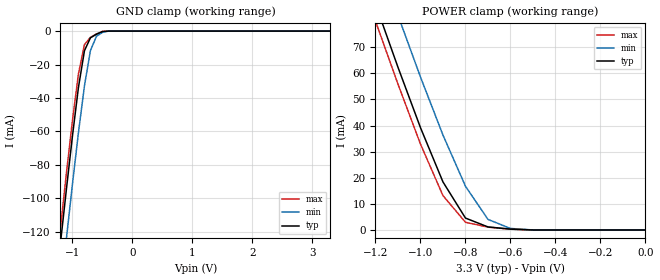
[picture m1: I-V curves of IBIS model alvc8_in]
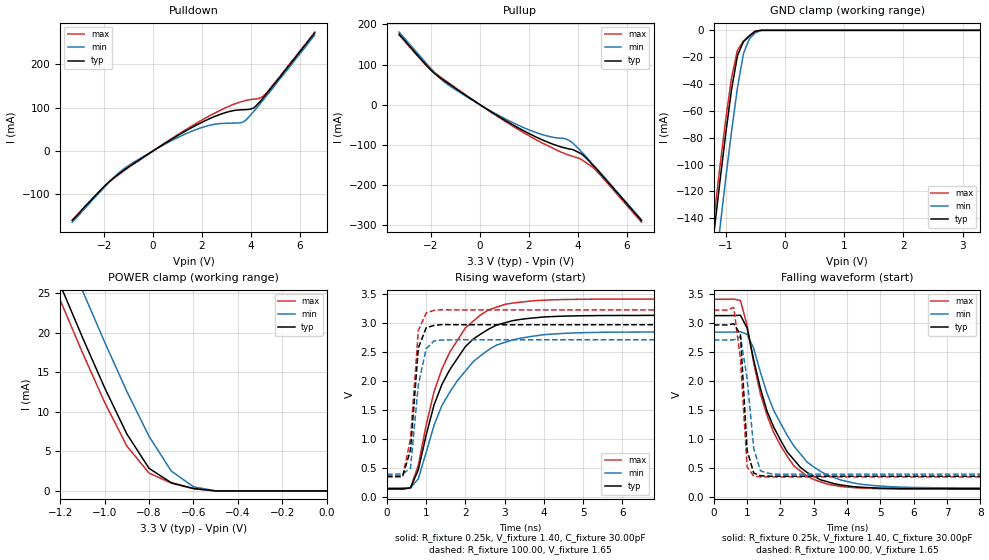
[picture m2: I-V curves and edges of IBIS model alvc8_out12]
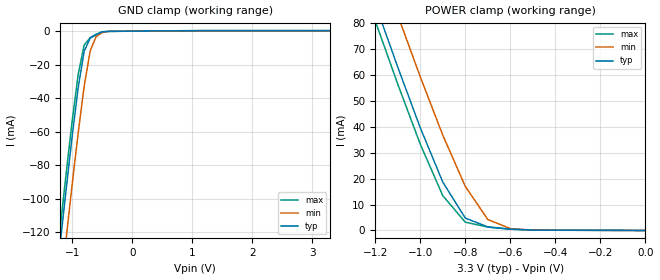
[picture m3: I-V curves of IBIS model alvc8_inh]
| IBIS file 162244ah.ibs created by s2ibis2 version 1.1
| North Carolina State University Electronics Research Laboratory  1995
[IBIS ver]   2.1
[File name]   162244ah.ibs
[File Rev]   1.0
[Date]   03/01/99 rtk rtk
[Source]   Integrated Device Technology, Inc.
[Notes]   1.Temperatures: typ=25C, min=100C, max=0C 2.RRmp rates based
   on 50 ohm load.
[Disclaimer] Integrated Device Technology, Inc. ("IDT") hereby grants the
   user of this IBIS model a non-exclusive, nontransferable
   license to use this IBIS model under the following terms. The
   user is granted this license only to use the IBIS model and is
   not granted rights to sell, copy (except as needed to run the
   IBIS model), rent, lease or sub-license the IBIS model in
   whole or in part, or in modified form to anyone. The User may
   modify the IBIS model to suit its specific applications, but
   rights to derivative works and such modifications shall belong
   to IDT. This IBIS model is provided on an AS IS" basis and IDT
   makes absolutely no warranty with respect to the information
   contained herein. IDT DISCLAIMS AND CUSTOMER WAIVES ALL
   WARRANTIES, EXPRESS AND IMPLIED, INCLUDING WARRANTIES OF
   MERCHANTABILITY AND FITNESS FOR A PARTICULAR PURPOSE. THE
   ENTIRE RISK AS TO QUALITY AND PERFORMANCE IS WITH THE USER
   ACCORDINGLY, IN NO EVENT SHALL IDT BE LIABLE FOR ANY DIRECT OR
   INDIRECT DAMAGES, WHETHER IN CONTRACT OR TORT, INCLUDING ANY
   LOST PROFITS OR OTHER INCIDENTAL, CONSEQUENTIAL, EXEMPLARY, OR
   PUNITIVE DAMAGES ARISING OUT OF THE USE OR APPLICATION OF THE
   IBIS model. Further, IDT reserves the right to make changes
   without notice to any product herein to improve reliability,
   function, or design. IDT does not convey any license under
   patent rights or any other intellectual property rights,
   including those of third parties. IDT is not obligated to
   provide maintenance or support for the licensed IBIS model.
[Copyright]   Copyright 1997, Integrated Device Technology, Inc. all rights
   reserved
|   Component ALVCH 162244
[Component]   ALVCH162244
[Manufacturer]   Integrated Device Technology
[Package]
| PA48
| variable   typ   min   max
R_pkg   6.50m   5.00m   10.00m
L_pkg   3.20nH   2.50nH   4.40nH
C_pkg   0.27pF   0.01pF   0.98pF
| PV48   typ   min   max
|R_pkg   6.5m   5.00m   10.00m
|L_pkg   4.75nH   3.82nH   6.72nH
|C_pkg   0.24pF   0.01pF   1.55pF
[Pin]  signal_name   model_name   R_pin   L_pin   C_pin
1   1OEB   alvc8_in
2   1Y1   alvc8_out12
3   1Y2   alvc8_out12
4   GND   GND
5   1Y3   alvc8_out12
6   1Y4   alvc8_out12
7   VCC   POWER
8   2Y1   alvc8_out12
9   2Y2   alvc8_out12
10   GND   GND
11   2Y3   alvc8_out12
12   2Y4   alvc8_out12
13   3Y1   alvc8_out12
14   3Y2   alvc8_out12
15   GND   GND
16   3Y3   alvc8_out12
17   3Y4   alvc8_out12
18   VCC   POWER
19   4Y1   alvc8_out12
20   4Y2   alvc8_out12
21   GND   GND
22   4Y3   alvc8_out12
23   4Y4   alvc8_out12
24   4OEB   alvc8_in
25   3OEB   alvc8_in
26   4A4   alvc8_inh
27   4A3   alvc8_inh
28   GND   GND
29   4A2   alvc8_inh
30   4A1   alvc8_inh
31   VCC   POWER
32   3A4   alvc8_inh
33   3A3   alvc8_inh
34   GND   GND
35   3A2   alvc8_inh
36   3A1   alvc8_inh
37   2A4   alvc8_inh
38   2A3   alvc8_inh
39   GND   GND
40   2A2   alvc8_inh
41   2A1   alvc8_inh
42   VCC   POWER
43   1A4   alvc8_inh
44   1A3   alvc8_inh
45   GND   GND
46   1A2   alvc8_inh
47   1A1   alvc8_inh
48   2OEB   alvc8_in
| Models and submodels in the file (3): alvc8_in (Input), alvc8_out12 (3-state), alvc8_inh (Input)
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| in   in   dummy_model
| oe   oe   dummy_model
|   Model alvc8_in
[Model]   alvc8_in
Model_type   Input
Vinl =  0.800V
Vinh =  2.000V
C_comp   3.00pF   NA   NA
[Temperature Range]   25.00   100.00   0.000
[Voltage Range]   3.30V   3.00V   3.60V
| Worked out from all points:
|   GND clamp passes 1 mA (typ) near -0.54 V on its own axis
|   POWER clamp passes 1 mA (typ) near -0.68 V on its own axis
[GND_clamp]
| voltage   I(typ)   I(min)   I(max)
-3.3V     -860mA     -887mA     -851mA
-1.3V     -161mA     -190mA     -151mA
-1.2V     -127mA     -157mA     -118mA
-1.1V     -94.41mA   -124mA     -84.85mA
-1V       -62.78mA   -91.54mA   -53.52mA
-900mV    -33.71mA   -60.78mA   -25.6mA
-800mV    -11.74mA   -32.83mA   -8.09mA
-700mV    -4.033mA   -11.65mA   -3.7mA
-600mV    -1.899mA   -3.108mA   -1.699mA
-500mV    -308uA     -810uA     -172uA
-400mV    -3.848nA   -9.872uA   -399pA
3.3V      39.6pA     19.33nA    26.4pA
[POWER_clamp]
| voltage   I(typ)   I(min)   I(max)
-3.3V     630mA      648mA      624mA
-1.2V     86.56mA    106mA      80.02mA
-1.1V     62.33mA    82.22mA    55.88mA
-1V       39.2mA     58.61mA    32.91mA
-900mV    18.4mA     36.35mA    13.15mA
-800mV    4.556mA    16.76mA    2.954mA
-700mV    1.164mA    4.056mA    1.087mA
-600mV    320uA      578uA      299uA
-500mV    40.08nA    12.23uA    3.465nA
0V        39.6pA     59.11pA    43.2pA
|   Model alvc8_out12
[Model]   alvc8_out12
Model_type   3-state
Polarity   Non-Inverting
Enable   Active-High
Vmeas =  1.500V
C_comp   3.00pF   NA   NA
[Temperature Range]   25.00   100.00   0.000
[Voltage Range]   3.30V   3.00V   3.60V
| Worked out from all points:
|   slope of the pulldown table from 0 to 0.495 V, typ, clamps not added: 27.6 ohm
|   slope of the pullup table from 0 to 0.495 V, typ, clamps not added: 25.8 ohm
|   GND clamp passes 1 mA (typ) near -0.51 V on its own axis
|   POWER clamp passes 1 mA (typ) near -0.69 V on its own axis
|   rising waveform, R_fixture 0.25k, V_fixture 1.40, C_fixture 30.00pF: 20-80 % time 1.05ns typ, 1.2ns min, 980ps max; typ from 0.138 V to 3.12 V
|   rising waveform, R_fixture 100.00, V_fixture 1.65: 20-80 % time 178ps typ, 250ps min, 201ps max; typ from 0.356 V to 2.96 V
|   falling waveform, R_fixture 0.25k, V_fixture 1.40, C_fixture 30.00pF: 20-80 % time 1.12ns typ, 1.35ns min, 1.05ns max; typ from 3.12 V to 0.138 V
|   falling waveform, R_fixture 100.00, V_fixture 1.65: 20-80 % time 157ps typ, 252ps min, 217ps max; typ from 2.96 V to 0.356 V
[Pulldown]
| voltage   I(typ)   I(min)   I(max)
-3.3V     -161mA     -165mA     -160mA
-1.8V     -71.5mA    -73.3mA    -72.6mA
-1.3V     -49.1mA    -46.1mA    -50.8mA
-600mV    -22.1mA    -19.8mA    -23.1mA
800mV     28.5mA     25mA       30mA
1.9V      63.5mA     52.4mA     68.3mA
3V        89.4mA     63.9mA     101mA
3.7V      95.4mA     67.5mA     115mA
4.1V      99.1mA     90.7mA     120mA
4.4V      116mA      111mA      123mA
4.6V      130mA      125mA      132mA
6.6V      273mA      268mA      275mA
[Pullup]
| voltage   I(typ)   I(min)   I(max)
-3.3V     176mA      181mA      174mA
-1.9V     80.3mA     83.6mA     82mA
-1.5V     61.8mA     58.9mA     64.3mA
-1V       40.8mA     37.7mA     42.5mA
400mV     -15.6mA    -14.2mA    -16.4mA
1.7V      -62.2mA    -54.9mA    -66.6mA
2.9V      -96.6mA    -80.2mA    -106mA
3.5V      -108mA     -85.3mA    -123mA
3.8V      -112mA     -96mA      -129mA
4.2V      -125mA     -121mA     -139mA
4.7V      -156mA     -155mA     -161mA
6.6V      -289mA     -287mA     -293mA
[GND_clamp]
| voltage   I(typ)   I(min)   I(max)
-3.3V     -1.007A    -1.04A     -997mA
-1.3V     -191mA     -226mA     -180mA
-1.2V     -152mA     -187mA     -141mA
-1.1V     -114mA     -149mA     -103mA
-1V       -77.54mA   -111mA     -67.03mA
-900mV    -44.06mA   -75.31mA   -35.25mA
-800mV    -18.73mA   -42.66mA   -14.81mA
-700mV    -8.526mA   -17.61mA   -7.964mA
-600mV    -4.327mA   -6.305mA   -3.891mA
-500mV    -756uA     -1.886mA   -436uA
-400mV    -8.73nA    -25.29uA   -695pA
3.3V      92.41pA    19.42nA    79.2pA
[POWER_clamp]
| voltage   I(typ)   I(min)   I(max)
-3.3V     175mA      181mA      173mA
-1.3V     32.91mA    38.88mA    30.95mA
-1.2V     26.11mA    32.08mA    24.16mA
-1.1V     19.45mA    25.38mA    17.52mA
-1V       13.07mA    18.85mA    11.22mA
-900mV    7.211mA    12.6mA     5.686mA
-800mV    2.858mA    6.904mA    2.259mA
-700mV    1.039mA    2.515mA    986uA
-600mV    306uA      524uA      278uA
-500mV    40.14nA    12.11uA    3.53nA
0V        92.41pA    138pA      101pA
[Ramp]
| variable   typ   min   max
dV/dt_r   1.29/0.24n   1.13/0.30n   1.44/0.25n
dV/dt_f   1.26/0.26n   1.08/0.26n   1.40/0.24n
R_load = 50.00
[Rising Waveform]
R_fixture = 0.25k
V_fixture = 1.40
C_fixture = 30.00pF
R_dut = 7.00m
L_dut = 3.30nH
C_dut = 0.29pF
| time   V(typ)   V(min)   V(max)
0s        138mV      152mV      132mV
600ps     154mV      154mV      155mV
800ps     468mV      312mV      549mV
1.2ns     1.581V     1.23V      1.809V
1.6ns     2.187V     1.801V     2.489V
2ns       2.587V     2.166V     2.908V
2.2ns     2.717V     2.327V     3.025V
3ns       2.995V     2.658V     3.313V
5.4ns     3.121V     2.832V     3.404V
19.8ns    3.124V     2.839V     3.405V
[Rising Waveform]
R_fixture = 100.00
V_fixture = 1.65
R_dut = 7.00m
L_dut = 3.30nH
C_dut = 0.29pF
| time   V(typ)   V(min)   V(max)
0s        356mV      391mV      343mV
400ps     356mV      392mV      344mV
600ps     806mV      494mV      1V
800ps     2.563V     1.932V     2.866V
1ns       2.912V     2.55V      3.166V
1.2ns     2.951V     2.684V     3.21V
1.4ns     2.965V     2.7V       3.222V
1.8ns     2.963V     2.704V     3.218V
19.8ns    2.963V     2.704V     3.218V
[Falling Waveform]
R_fixture = 0.25k
V_fixture = 1.40
C_fixture = 30.00pF
R_dut = 7.00m
L_dut = 3.30nH
C_dut = 0.29pF
| time   V(typ)   V(min)   V(max)
0s        3.124V     2.839V     3.405V
800ps     3.13V      2.846V     3.383V
1ns       2.909V     2.8V       2.955V
1.2ns     2.353V     2.557V     2.296V
1.4ns     1.866V     2.145V     1.771V
1.8ns     1.2V       1.489V     1.106V
2.4ns     642mV      879mV      534mV
3.4ns     261mV      376mV      220mV
5.8ns     142mV      164mV      135mV
19.8ns    138mV      152mV      132mV
[Falling Waveform]
R_fixture = 100.00
V_fixture = 1.65
R_dut = 7.00m
L_dut = 3.30nH
C_dut = 0.29pF
| time   V(typ)   V(min)   V(max)
0s        2.963V     2.704V     3.218V
400ps     2.963V     2.704V     3.218V
600ps     2.983V     2.705V     3.264V
800ps     2.795V     2.761V     2.38V
1ns       801mV      2.038V     518mV
1.2ns     409mV      830mV      356mV
1.4ns     364mV      449mV      345mV
1.6ns     357mV      410mV      343mV
1.8ns     356mV      390mV      343mV
19.8ns    356mV      391mV      343mV
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|   Model alvc8_inh
[Model]   alvc8_inh
Model_type   Input
Vinl =  0.800V
Vinh =  2.000V
C_comp   3.00pF   NA   NA
[Temperature Range]   25.00   100.00   0.000
[Voltage Range]   3.30V   3.00V   3.60V
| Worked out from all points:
|   GND clamp passes 1 mA (typ) near -0.53 V on its own axis
|   POWER clamp passes 1 mA (typ) near -0.66 V on its own axis
[GND_clamp]
| voltage   I(typ)   I(min)   I(max)
-3.3V     -860mA     -888mA     -852mA
-1.3V     -161mA     -190mA     -151mA
-1.2V     -127mA     -157mA     -118mA
-1.1V     -94.51mA   -124mA     -84.99mA
-1V       -62.91mA   -91.62mA   -53.71mA
-900mV    -33.88mA   -60.87mA   -25.82mA
-800mV    -11.92mA   -32.93mA   -8.306mA
-700mV    -4.211mA   -11.77mA   -3.908mA
-600mV    -2.051mA   -3.213mA   -1.882mA
-500mV    -472uA     -914uA     -379uA
-400mV    -144uA     -112uA     -169uA
3.3V      264uA      163uA      349uA
[POWER_clamp]
| voltage   I(typ)   I(min)   I(max)
-3.3V     638mA      656mA      632mA
-1.2V     87.67mA    108mA      81.05mA
-1.1V     63.19mA    83.28mA    56.62mA
-1V       39.75mA    59.43mA    33.41mA
-900mV    18.73mA    36.86mA    13.47mA
-800mV    4.8mA      17.05mA    3.222mA
-700mV    1.374mA    4.243mA    1.32mA
-600mV    498uA      728uA      497uA
-500mV    146uA      134uA      162uA
0V        45.19pA    64.49pA    49.16pA
